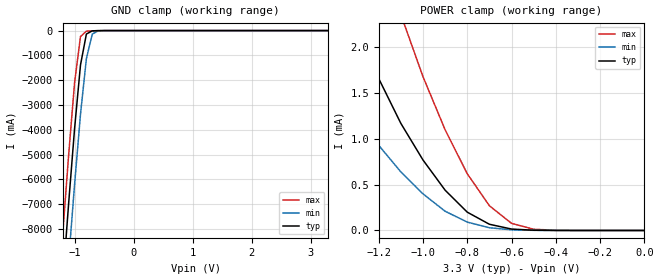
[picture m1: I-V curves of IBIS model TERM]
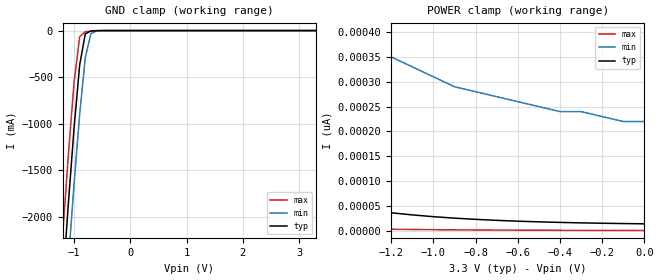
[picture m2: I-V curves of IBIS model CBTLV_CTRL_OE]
| I/O Buffer Information Specification (IBIS) Version 3.2 (August 20, 1999)
| IBIS is a standard for electronic behavioral specifications of integrated
| circuit input/output analog characteristics.
[IBIS Ver]   3.2
[File Name]   cbtlv3862.ibs
[File Rev]   1.1
[Date]   Tuesday, October 16 2001
[Source]   Integrated Device Technology, Inc.
[Notes]   1.Temperatures: typ=25C, min=-40C, max=100C
[Disclaimer] Integrated Device Technology, Inc. ("IDT") hereby grants the
   user of this IBIS model a non-exclusive, nontransferable
   license to use this IBIS model under the following terms. The
   user is granted this license only to use the IBIS model and is
   not granted rights to sell, copy (except as needed to run the
   IBIS model), rent, lease or sub-license the IBIS model in
   whole or in part, or in modified form to anyone. The User may
   modify the IBIS model to suit its specific applications, but
   rights to derivative works and such modifications shall belong
   to IDT.
   This IBIS model is provided on an AS IS" basis and IDT
   makes absolutely no warranty with respect to the information
   contained herein. IDT DISCLAIMS AND CUSTOMER WAIVES ALL
   WARRANTIES, EXPRESS AND IMPLIED, INCLUDING WARRANTIES OF
   MERCHANTABILITY AND FITNESS FOR A PARTICULAR PURPOSE. THE
   ENTIRE RISK AS TO QUALITY AND PERFORMANCE IS WITH THE USER
   ACCORDINGLY, IN NO EVENT SHALL IDT BE LIABLE FOR ANY DIRECT OR
   INDIRECT DAMAGES, WHETHER IN CONTRACT OR TORT,  INCLUDING
   ANY LOST PROFITS OR OTHER INCIDENTAL, CONSEQUENTIAL, EXEMPLARY,
   OR PUNITIVE DAMAGES ARISING OUT OF THE USE OR APPLICATION OF
   THE IBIS model.
   Further, IDT reserves the right to make changes without notice
   to any product herein to improve reliability, function, or
   design. IDT does not convey any license under patent rights or
   any other intellectual property rights, including those of
   third parties. IDT is not obligated to provide maintenance or
   support for the licensed IBIS model.
[Copyright]   Copyright 1997, Integrated Device Technology, Inc. all rights
   reserved
|   Component IDT74CBTLV3862
[Component]   IDT74CBTLV3862
[Manufacturer]   Integrated Device Technology
[Package]
|Following package parameters are for SSOP 24 lead package
| variable   typ   min   max
R_pkg   4.00m   2.00m   5.00m
L_pkg   5.01nH   4.65nH   6.05nH
C_pkg   0.045pF   0.035pF   0.067pF
[Pin]  signal_name   model_name   R_pin   L_pin   C_pin
1   OE   CBTLV_CTRL_OE
2   A1   TERM
3   A2   TERM
4   A2   TERM
5   A4   TERM
6   A5   TERM
7   A6   TERM
8   A7   TERM
9   A8   TERM
10   A9   TERM
11   A10   TERM
12   GND   GND
13   B10   TERM
14   B9   TERM
15   B8   TERM
16   B7   TERM
17   B6   TERM
18   B5   TERM
19   B4   TERM
20   B3   TERM
21   B2   TERM
22   B1   TERM
23   _OE_   CBTLV_CTRL_OEB
24   VCC   POWER
| oeb  oeb   dummy_model
[Series Switch Groups]
|Function Group States
On A /
Off A /
[Series Pin Mapping]   pin_2   model_name   function_table_group
2   22   CBTLV_SW   A
3   21   CBTLV_SW   A
4   20   CBTLV_SW   A
5   19   CBTLV_SW   A
6   18   CBTLV_SW   A
7   17   CBTLV_SW   A
8   16   CBTLV_SW   A
9   15   CBTLV_SW   A
10   14   CBTLV_SW   A
11   13   CBTLV_SW   A
|   Model CBTLV_SW
[Model]   CBTLV_SW
Model_type   Series_switch
C_comp   0.00pF   0.00pF   0.00pF
[Temperature Range]   25.00   100.00   -40.00
[Voltage Range]   3.30V   3.00V   3.6V
[On]
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[Off]
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| Models and submodels in the file (4): TERM (Terminator), CBTLV_CTRL_OE (Input), CBTLV_CTRL_OEB (Input), CBTLV_SW (Series_switch)
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|   Model TERM
[Model]   TERM
Model_type   Terminator
Polarity   Non-Inverting
C_comp   5.00pF   5.00pF   5.00pF
[Temperature Range]   25.00   100.00   -40.00
[Voltage Range]   3.30V   3.00V   3.60V
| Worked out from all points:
|   GND clamp passes 1 mA (typ) near -0.54 V on its own axis
|   POWER clamp passes 1 mA (typ) near -1.06 V on its own axis
[GND_clamp]
| voltage   I(typ)   I(min)   I(max)
-3.3V     -82.19A    -84.14A    -80.6A
-1.2V     -10.13A    -12.44A    -8.17A
-1.1V     -6.95A     -9.26A     -5A
-1V       -3.95A     -6.2A      -2.1A
-900mV    -1.39A     -3.38A     -240mA
-800mV    -140mA     -1.13A     -23mA
-700mV    -10.38mA   -140mA     -11.02mA
-600mV    -2.14mA    -10.9mA    -3.97mA
3.3V      43.59pA    38.63nA    59.54pA
[POWER_clamp]
| voltage   I(typ)   I(min)   I(max)
-3.3V     19.83mA    14.03mA    24.7mA
-1.6V     4.15mA     2.52mA     6.59mA
-1.5V     3.45mA     2.06mA     5.66mA
-1.3V     2.2mA      1.26mA     3.9mA
-1.1V     1.17mA     640uA      2.36mA
-1V       770uA      400uA      1.68mA
-900mV    440uA      210uA      1.1mA
-800mV    200uA      91.79uA    620uA
-700mV    67.88uA    29.64uA    270uA
-600mV    15.52uA    7.26uA     77.81uA
-500mV    2.7uA      1.47uA     13.43uA
0V        43.57pA    640pA      91.39pA
|   Model CBTLV_CTRL_OE
[Model]   CBTLV_CTRL_OE
Model_type   Input
Vinl =   0.80V
Vinh =   2.00V
C_comp   5.00pF   5.00pF   5.00pF
[Temperature Range]   25.00   100.00   -40.00
[Voltage Range]   3.30V   3.00V   3.60V
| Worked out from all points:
|   GND clamp passes 1 mA (typ) near -0.58 V on its own axis
[GND_clamp]
| voltage   I(typ)   I(min)   I(max)
-3.3V     -22A       -22.54A    -21.56A
-1.2V     -2.71A     -3.33A     -2.18A
-1.1V     -1.85A     -2.47A     -1.33A
-1V       -1.05A     -1.65A     -560mA
-900mV    -370mA     -900mA     -66.52mA
-800mV    -35.18mA   -290mA     -11.47mA
-700mV    -4.02mA    -32.89mA   -5.96mA
-600mV    -1.16mA    -2.31mA    -2.17mA
3.3V      14.11pA    240pA      630fA
[POWER_clamp]
| voltage   I(typ)   I(min)   I(max)
-3.3V     620pA      3.78nA     60.89pA
-3V       430pA      2.65nA     42.48pA
-2.9V     380pA      2.34nA     37.5pA
-2.6V     260pA      1.61nA     25.42pA
-2.3V     170pA      1.1nA      16.85pA
-2V       110pA      760pA      10.91pA
-1.8V     84.03pA    610pA      8.09pA
-1.4V     47.41pA    410pA      4.34pA
-1.2V     36.31pA    350pA      3.19pA
-900mV    25.54pA    290pA      2.02pA
-400mV    16.97pA    240pA      1.06pA
0V        14.1pA     220pA      750fA
